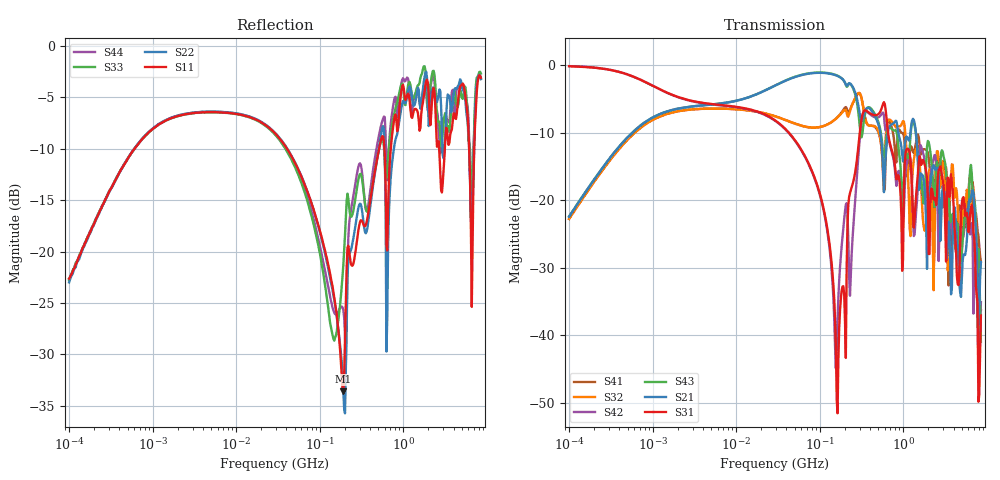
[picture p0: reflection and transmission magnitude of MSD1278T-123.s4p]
# MHz S MA R 50
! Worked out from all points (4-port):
!   498 points, 100 kHz to 8.5 GHz, reference 50 ohm
!   strongest paths, dB at 100 kHz, 1.698 MHz, 29.49 MHz, 500.7 MHz, 8.5 GHz:
!     S31: -0.1, -4.4, -8.2, -7.3, -37.1
!     S21: -22.5, -6.6, -3.0, -8.7, -29.2
!     S43: -22.4, -6.7, -3.0, -8.3, -41.0
!     S42: -0.1, -4.4, -8.3, -7.7, -35.1
!     S32: -22.8, -7.0, -7.6, -9.7, -36.3
!     S41: -22.7, -7.0, -7.6, -9.8, -29.1
!   lowest |S11| = -33.6 dB at 191.9 MHz (marker M1), VSWR 1.04, Z = 52.1 - j0.216 ohm
!   |S11| at or under -10 dB: 40.66 MHz to 513.7 MHz (473 MHz wide, 171 % of centre); 2.687 GHz to 3.147 GHz (459.4 MHz wide, 15.7 % of centre); 6.148 GHz to 7.071 GHz (923.8 MHz wide, 14 % of centre)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
0.1  0.0739 78.4  0.0754 79.5  0.9834 -4.3  0.07287 -101.1
     0.0754 79.5  0.07084 79.8  0.07274 -101.0  0.984 -4.4
     0.9834 -4.3  0.07274 -101.0  0.07256 79.5  0.07598 79.2
     0.07287 -101.1  0.984 -4.4  0.07598 79.2  0.07348 80.4
15.91744  0.4455 -21.7  0.5946 13.7  0.4643 -28.5  0.457 152.2
          0.5946 13.7  0.4479 -22.1  0.458 151.7  0.461 -28.5
          0.4643 -28.5  0.458 151.7  0.4426 -22.3  0.5955 13.7
          0.457 152.2  0.461 -28.5  0.5955 13.7  0.446 -21.7
156.2097  0.05288 -70.4  0.842 -39.1  0.008065 -129.1  0.4024 46.6
          0.842 -39.1  0.05153 -75.7  0.4005 45.2  0.005687 159.0
          0.008065 -129.1  0.4005 45.2  0.03905 -4.4  0.8463 -41.5
          0.4024 46.6  0.005687 159.0  0.8463 -41.5  0.04988 -25.3
191.855  0.02086 -5.7  0.7767 -51.7  0.02309 42.4  0.4669 31.1
         0.7767 -51.7  0.021 -87.7  0.4574 29.2  0.06263 55.8
         0.02309 42.4  0.4574 29.2  0.08634 35.8  0.7771 -55.3
         0.4669 31.1  0.06263 55.8  0.7771 -55.3  0.05193 -4.9
587.4518  0.3436 -27.1  0.1148 -92.0  0.5327 -85.1  0.1323 -79.9
          0.1148 -92.0  0.3873 -49.3  0.1188 -53.0  0.4236 -92.0
          0.5327 -85.1  0.1188 -53.0  0.324 -7.3  0.1862 -99.7
          0.1323 -79.9  0.4236 -92.0  0.1862 -99.7  0.4539 -7.0
2209.207  0.5425 -173.7  0.1653 142.3  0.1214 143.0  0.121 88.2
          0.1653 142.3  0.6094 -171.9  0.09252 84.1  0.181 126.5
          0.1214 143.0  0.09252 84.1  0.7274 179.0  0.1739 114.2
          0.121 88.2  0.181 126.5  0.1739 114.2  0.6932 -177.6
8500  0.7012 -53.6  0.03486 -30.9  0.01402 -28.8  0.03496 -170.9
      0.03486 -30.9  0.6904 -56.9  0.01535 -152.9  0.01755 -29.0
      0.01402 -28.8  0.01535 -152.9  0.7352 -48.2  0.008911 -101.7
      0.03496 -170.9  0.01755 -29.0  0.008911 -101.7  0.6952 -52.0
